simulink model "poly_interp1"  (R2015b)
settings: Solver=VariableStepAuto  StartTime=0.0  StopTime=15  RelTol=1e-3
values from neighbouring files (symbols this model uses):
  g = firpolyphase(hdez, M)    [poly_dez_1.m]    (also in poly_dez_2.m; poly_interp_1.m = firpolyphase(hint, L); poly_interp_2.m = firpolyphase(hint, L))
  hint = fir1(nord, 0.9*1/L)    [interpol_1.m]    (also in interpol_2.m = fir1(nord, 1/L); poly_interp_1.m = fir1(nord2, 1/L); poly_interp_2.m = fir1(nord2, 1/L))
  hTP = fir1(nord, 2*fp/fs)    [dezimier_2.m]    (also in dezimier_3.m; frac_delay_1.m = fir1(nord, fp*2); frac_delay_2.m = fir1(nord, fp*2); lagrange_3.m = fir1(40, 0.5))
  L = 3    [farrow_3.m]    (also in farrow_4.m = 480; ifir_1.m = 5; ifir_dezim_1.m = 5; ifir_high1.m = 5)
  Ts = 1/fs    (= 5e-05)    [basisband_1.m]    (also in basisband_2.m = 5e-06; dezimier_1.m = 0.0005; dezimier_11.m = 0.0005; dezimier_2.m = 0.0005)
libraries: dspsigops x5, simulink x1, dspmlti4 x1

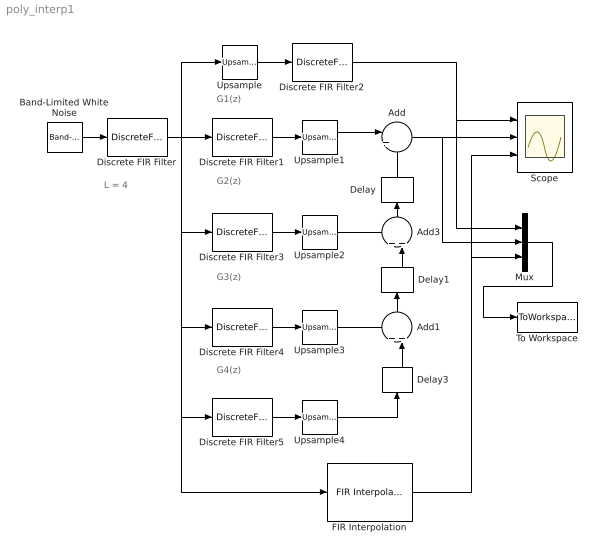
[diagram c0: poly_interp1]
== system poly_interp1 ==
  note: G1(z)
  note: G2(z)
  note: G3(z)
  note: G4(z)
  note: L = 4
  Add : Sum  Inputs=|++
  Add1 : Sum  Inputs=++|
  Add3 : Sum  Inputs=++|
  Band-Limited White Noise : simulink/Sources/Band-Limited White Noise  Cov=Ts  Ts=Ts  seed=[23341]
  Delay : Delay  DelayLength=1
  Delay1 : Delay  DelayLength=1
  Delay3 : Delay  DelayLength=1
  Discrete FIR Filter : DiscreteFir  Coefficients=hTP
  Discrete FIR Filter1 : DiscreteFir  Coefficients=(g(1,:))
  Discrete FIR Filter2 : DiscreteFir  Coefficients=hint
  Discrete FIR Filter3 : DiscreteFir  Coefficients=(g(2,:))
  Discrete FIR Filter4 : DiscreteFir  Coefficients=(g(3,:))
  Discrete FIR Filter5 : DiscreteFir  Coefficients=(g(4,:))
  FIR Interpolation : dspmlti4/FIR Interpolation  FilterSource=Dialog parameters  h=hint  L=4  FilterObject=Hm_firinterp  InputProcessing=Columns as channels (frame based)  framing=Allow multirate processing  outputBufInitCond=0  roundingMode=Floor  overflowMode=off  firstCoeffDataTypeStr=Inherit: Same word length as input  firstCoeffMin=[]  firstCoeffMax=[]  firstCoeffLastDataTypeStr=Inherit: Same word length as input  outputDataTypeStr=Inherit: Same as accumulator  outputMin=[]  outputMax=[]  outputLastDataTypeStr=Inherit: Same as accumulator
  Mux : Mux  Inputs=3
  Scope : Scope  NumInputPorts=3
  To Workspace : ToWorkspace  VariableName=y  SaveFormat=Timeseries  SampleTime=-1
  Upsample{,1..4} (5 alike) : dspsigops/Upsample  N=L  phase=0  RateOptions=Allow multirate processing  ic=0  mode=Unused parameter value
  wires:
  Band-Limited White Noise/1 -> Discrete FIR Filter/1
  Discrete FIR Filter1/1 -> Upsample1/1
  Discrete FIR Filter3/1 -> Upsample2/1
  Discrete FIR Filter4/1 -> Upsample3/1
  Discrete FIR Filter5/1 -> Upsample4/1
  Discrete FIR Filter2/1 -> Mux/1, Scope/1
  FIR Interpolation/1 -> Mux/3, Scope/3
  Discrete FIR Filter/1 -> Discrete FIR Filter1/1, Upsample/1, FIR Interpolation/1, Discrete FIR Filter5/1, Discrete FIR Filter4/1, Discrete FIR Filter3/1
  Upsample/1 -> Discrete FIR Filter2/1
  Upsample1/1 -> Add/1
  Add/1 -> Mux/2, Scope/2
  Upsample2/1 -> Add3/1
  Add3/1 -> Delay/1
  Delay/1 -> Add/2
  Upsample3/1 -> Add1/1
  Upsample4/1 -> Delay3/1
  Delay3/1 -> Add1/2
  Mux/1 -> To Workspace/1
  Add1/1 -> Delay1/1
  Delay1/1 -> Add3/2
